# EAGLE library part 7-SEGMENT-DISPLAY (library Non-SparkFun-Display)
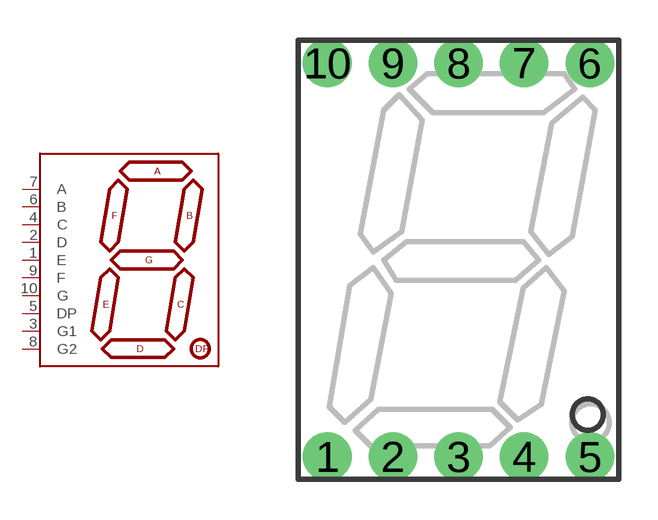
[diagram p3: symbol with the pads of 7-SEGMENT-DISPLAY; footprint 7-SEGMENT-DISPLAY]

Designator prefix -

## 7-SEGMENT-DISPLAYPTH  [7-SEGMENT-DISPLAY]
1  E
2  D
3  G1
4  C
5  DP
6  B
7  A
8  G2
9  F
10  G

## Footprint 7-SEGMENT-DISPLAY (pad centres in mm)
drill 0.65 pad 1.88: 1 -5.08,-7.62; 2 -2.54,-7.62; 3 0,-7.62; 4 2.54,-7.62; 5 5.08,-7.62; 6 5.08,7.62; 7 2.54,7.62; 8 0,7.62; 9 -2.54,7.62; 10 -5.08,7.62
